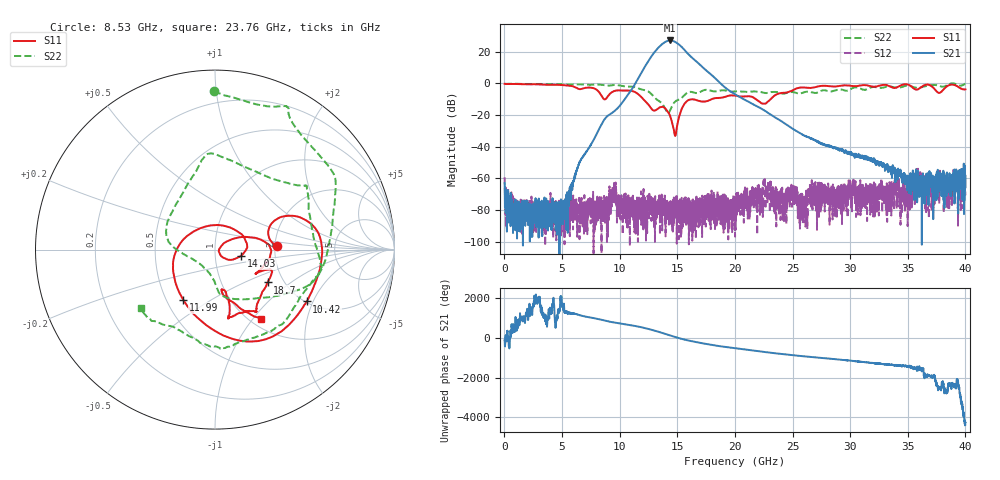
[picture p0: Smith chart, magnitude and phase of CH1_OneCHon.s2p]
!Keysight Technologies,N5245B,MY57181321,A.14.80.03
!Date: Thursday, August 24, 2023 17:11:17
!Correction: S11(C  2-Port  )
!S21(C  2-Port  )
!S12(C  2-Port  )
!S22(C  2-Port  )
!S2P File: Measurements: S11, S21, S12, S22:
# Hz S  RI  R 50
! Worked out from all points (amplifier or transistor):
!   4000 points, 10 MHz to 40 GHz, reference 50 ohm
!   highest |S21| = 27.1 dB at 14.38 GHz (marker M1)
!   |S21| within 3 dB of that: 13.57 GHz to 15.21 GHz (1.64 GHz wide, 11.4 % of centre)
!   unconditionally stable (mu >= 1): start of sweep to 38.84 GHz; 38.9 GHz to end of sweep
!   at 6.67 GHz: K = 336078.69, MAG = -37.3 dB, |S12| = -89.8 dB
!   at 20.01 GHz: K = 45687.62, MAG = -4.6 dB, |S12| = -96.9 dB
!   at 40 GHz: K = 94918.53, MAG = -50.1 dB, |S12| = -70.8 dB
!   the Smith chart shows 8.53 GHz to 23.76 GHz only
!   S11 on the Smith chart (normalised r, x): 8.53 GHz: 2.06, +0.09; 10.42 GHz: 2.03, -1.79; 11.99 GHz: 0.61, -0.38; 14.03 GHz: 1.33, -0.09; 18.7 GHz: 1.65, -0.69; 23.76 GHz: 1.12, -1.11
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1e7  -0.9564 0.0458  -0.000306 -0.00064  -0.000111 -0.00107  -0.9607 0.0229
6.68e9  0.3478 0.5649  0.00331 0.00251  0.000101 -6.05e-06  -0.3476 0.8484
8.53e9  0.3477 0.0182  -0.0598 0.00152  -0.000158 8.24e-05  -0.00614 0.8821
1.042e10  0.5111 -0.289  0.2605 -0.164  -4.64e-05 0.000147  0.5022 0.6134
1.199e10  -0.1768 -0.2797  -2.383 0.9176  1.06e-05 -0.00017  0.6249 -0.0175
1.276e10  -0.1206 0.1003  4.855 5.242  6.81e-05 0.000105  0.3785 -0.25
1.334e10  0.1216 0.1036  8.594 -10.01  -6.83e-05 9.51e-06  0.0833 -0.2729
1.37e10  0.1786 0.026  -6.736 -16.1  0.000177 6.94e-05  0.0159 -0.2247
1.403e10  0.1443 -0.0344  -20.79 -2.456  3.68e-05 5.16e-05  -0.0286 -0.1345
1.42e10  0.109 -0.0522  -19.97 9.416  8.87e-05 -5.65e-06  -0.0706 -0.0904
1.438e10  0.0722 -0.0559  -11.54 19.35  0.00017 -6.11e-05  -0.1329 -0.0482
1.464e10  0.0296 -0.0283  6.424 20.58  -4.73e-05 -2.29e-05  -0.2203 0.00431
1.499e10  0.0401 0.025  18.12 3.5  7.47e-05 -3.81e-05  -0.2727 0.1043
1.544e10  0.1575 0.0707  6.297 -11.76  1.54e-05 -6.23e-05  -0.18 0.3139
1.606e10  0.3032 0.0208  -6.281 -4.295  0.000197 -1.73e-05  -0.0401 0.5332
1.688e10  0.2547 -0.1099  -2.01 3.605  -3.66e-05 -0.000141  0.3122 0.3981
1.87e10  0.2926 -0.1831  0.5038 -0.9  -3.22e-05 8.69e-05  0.5841 -0.0548
2.001e10  0.2191 -0.3445  -0.4176 -0.1552  -4.25e-06 1.36e-05  0.411 -0.3697
2.376e10  0.2579 -0.3882  0.0205 -0.0697  0.000331 -7.05e-05  -0.4107 -0.3275
2.667e10  -0.114 -0.7104  -0.00743 0.016  -0.000454 0.000741  -0.3305 0.3971
3.334e10  -0.8274 0.0302  0.000129 0.00239  0.000101 -5.51e-05  0.7689 -0.1834
4e10  0.3062 0.5629  0.000147 0.00051  1.39e-06 -0.000289  0.2102 -0.952
